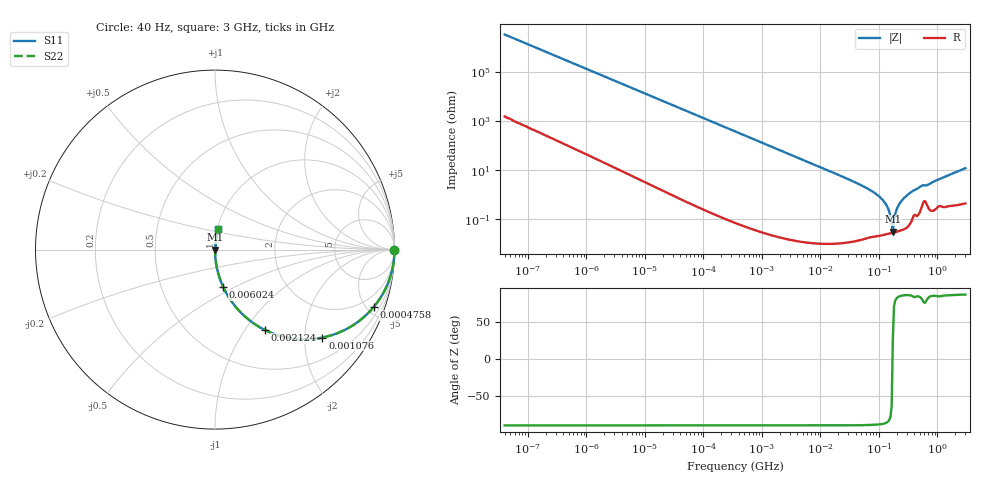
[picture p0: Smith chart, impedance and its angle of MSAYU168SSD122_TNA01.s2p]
! MSAYU168SSD122_TNA01  S-PARAMETER MODEL  ( General Type )
! Model Generated by TAIYO YUDEN Corporation (http://www.ty-top.com)
! Version 2.0
! TAIYO YUDEN Control No. 030711
! Copyright(c) 2003 TAIYO YUDEN CO.,LTD. All Rights Reserved.
! Product Description (link to TY-COMPAS)
! https://ds.yuden.co.jp/TYCOMPAS/or/detail?pn=MSAYU168SSD122KTNA01&u=M
! Products Name : Multilayer Ceramic Capacitors
! Characteristics :
!  Capacitance : 1200 pF , Rated Voltage : 50V
!  Case Size : 1.6 x 0.8 / 0.063 x 0.031 [mm/inch] , Thickness : 0.8 / 0.031 [mm/inch]
!  (Conditions: Temperature = 25 degC , DC Bias Current/Voltage = 0A / 0V)
! External Node Assignments :
!  1  o---| |---o  2
! GND o---------o GND
! Frequency Range : 40Hz  -  3GHz  [ 401 STEP ]
# MHz S RI R 50
! Freq[MHz].  S11 Real  S11 Imag  S21 Real  S21 Imag  S12 Real  S12 Imag  S22 Real  S22 Imag
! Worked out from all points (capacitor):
!   401 points, 40 Hz to 3 GHz, reference 50 ohm
!   read as one part in series: C = 1.21 nF near 44 Hz
!   lowest |Z| = 31.1 mohm at 172.5 MHz (marker M1)
!   series resonance near 171 MHz, so ESL is about 720 pH
!   S11 on the Smith chart (normalised r, x): 40 Hz: open; 475.8 kHz: 1.00, -5.52; 1.076 MHz: 1.00, -2.44; 2.124 MHz: 1.00, -1.24; 6.024 MHz: 1.00, -0.44; 3 GHz: 1.01, +0.24
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4e-05  1 -3.04e-05  1.5e-08 3.04e-05  1.5e-08 3.04e-05  1 -3.04e-05
0.000136  1 -0.000103  5.3e-08 0.000103  5.3e-08 0.000103  1 -0.000103
0.000834  1 -0.000635  6.18e-07 0.000635  6.18e-07 0.000635  1 -0.000635
0.017386  0.9998 -0.0132  0.000178 0.0132  0.000178 0.0132  0.9998 -0.0132
0.106589  0.9934 -0.0806  0.00655 0.0806  0.00655 0.0806  0.9934 -0.0806
0.362475  0.9293 -0.2563  0.0707 0.2563  0.0707 0.2563  0.9293 -0.2563
0.475778  0.8841 -0.3201  0.1159 0.3201  0.1159 0.3201  0.8841 -0.3201
1.075925  0.5986 -0.4901  0.4014 0.4901  0.4014 0.4901  0.5986 -0.4901
2.123718  0.2769 -0.4473  0.7231 0.4473  0.7231 0.4473  0.2769 -0.4473
6.024386  0.0454 -0.2079  0.9546 0.2079  0.9546 0.2079  0.0454 -0.2079
7.222098  0.032 -0.1758  0.968 0.1758  0.968 0.1758  0.032 -0.1758
76.28187  0.000379 -0.0138  0.9996 0.0138  0.9996 0.0138  0.000379 -0.0138
120.0322  0.000262 -0.00552  0.9997 0.00552  0.9997 0.00552  0.000262 -0.00552
137.5184  0.000262 -0.00336  0.9997 0.00336  0.9997 0.00336  0.000262 -0.00336
150.5692  0.000266 -0.00195  0.9997 0.00195  0.9997 0.00195  0.000266 -0.00195
157.552  0.00027 -0.00127  0.9997 0.00127  0.9997 0.00127  0.00027 -0.00127
172.504  0.000281 0.000133  0.9997 -0.000133  0.9997 -0.000133  0.000281 0.000133
180.504  0.000289 0.000847  0.9997 -0.000847  0.9997 -0.000847  0.000289 0.000847
226.4253  0.00036 0.00442  0.9996 -0.00442  0.9996 -0.00442  0.00036 0.00442
340.4975  0.000799 0.0119  0.9992 -0.0119  0.9992 -0.0119  0.000799 0.0119
535.7849  0.0036 0.0226  0.9964 -0.0226  0.9964 -0.0226  0.0036 0.0226
3000  0.0183 0.1169  0.9817 -0.1169  0.9817 -0.1169  0.0183 0.1169
